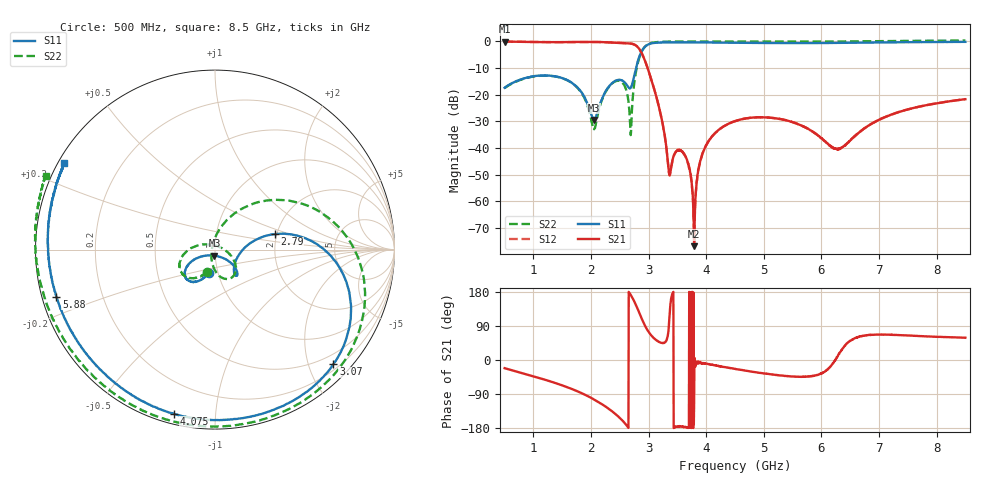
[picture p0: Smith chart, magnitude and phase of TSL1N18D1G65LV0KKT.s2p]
!TSL1N18D1G65LV0KKT  S-PARAMETER MODEL  ( General Type )
! Model Generated by TAIYO YUDEN Corporation (https://www.yuden.co.jp/en/)
! Version 1.0
! TAIYO YUDEN Control No. 240527
! Copyright(c) 2024 TAIYO YUDEN CO.,LTD. All Rights Reserved.
! Products Name : Ceramic RF Devices
! Characteristics :
!  Passband freq :617-2690MHz, , ( At Passband , Insertion Loss :1.35dB, VSWR 2.0 )
!  Attenuation :30 dB min at 3300 to 3800MHz,24 dB min at 4400to 7125MHz, Impedance : 50 Ohm
!  Case Size : 1.6 x 0.8 / 0.063 x 0.031 [mm/inch] , Thickness : 0.65 / 0.026 [mm/inch]
!  (Conditions: Temperature = 25 degC , DC Bias Current/Voltage = 0A / 0V)
! External Node Assignments :
!  1  o---|-------|---o  2
!  |  LPF  |
! GND o---|-------|---o GND
! Frequency Range : 500MHz  -  8.5GHz  [ 1601 STEP ]
# MHz S RI R 50
! Freq[MHz].  S11 Real  S11 Imag  S21 Real  S21 Imag  S12 Real  S12 Imag  S22 Real  S22 Imag
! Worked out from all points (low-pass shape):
!   1601 points, 500 MHz to 8.5 GHz, reference 50 ohm
!   highest |S21| = -0.15 dB at 500 MHz (marker M1); lowest = -76.8 dB at 3.79 GHz (marker M2)
!   |S21| within 3 dB of the highest: start of sweep to 2.845 GHz
!   lowest |S11| = -29.5 dB at 2.055 GHz (marker M3), VSWR 1.07, Z = 49.6 - j3.31 ohm
!   |S11| at or under -10 dB: start of sweep to 2.782 GHz
!   |S22| runs from -35.2 to 0.3 dB; largest |S21 - S12| = 0.0035
!   S11 on the Smith chart (normalised r, x): 500 MHz: 0.90, -0.24; 2.79 GHz: 1.95, +0.38; 3.07 GHz: 0.30, -2.44; 4.075 GHz: 0.05, -0.78; 5.88 GHz: 0.04, -0.14; 8.5 GHz: 0.02, +0.27
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500  -0.0351 -0.1294  0.9144 -0.3612  0.9142 -0.3619  -0.045 -0.1235
1280  -0.1622 -0.1571  0.5387 -0.7928  0.5377 -0.7915  -0.1935 -0.1141
1835  -0.0994 -0.0467  0.0446 -0.9672  0.0421 -0.9657  -0.1047 0.0206
2055  -0.00296 -0.0333  -0.2403 -0.938  -0.2411 -0.9365  0.00809 0.021
2430  0.1244 -0.1337  -0.7505 -0.5604  -0.7497 -0.5585  0.106 -0.1428
2580  0.1074 -0.1335  -0.8916 -0.2311  -0.8915 -0.2294  0.0239 -0.1471
2690  0.1305 -0.0342  -0.8932 0.1312  -0.8926 0.1331  -0.0172 0.00303
2790  0.3328 0.0864  -0.64 0.5042  -0.6389 0.5038  0.18 0.2417
2935  0.7481 -0.2366  -0.0102 0.436  -0.00937 0.4366  0.7859 -0.019
3070  0.6596 -0.6385  0.0773 0.1386  0.0779 0.1391  0.7712 -0.5324
3170  0.5185 -0.7863  0.0427 0.0483  0.0421 0.0489  0.6227 -0.7375
3355  0.2946 -0.904  -0.000484 0.00331  -0.000401 0.00336  0.3637 -0.9105
3615  0.0658 -0.9484  -0.00764 -0.000329  -0.00768 -0.000477  0.0948 -0.9799
3790  -0.059 -0.9475  -6.23e-05 -0.000131  9.43e-05 -0.000155  -0.0434 -0.985
3900  -0.1263 -0.938  0.00587 -0.00068  0.00579 -0.000702  -0.1179 -0.9784
4075  -0.2261 -0.9162  0.0147 -0.00325  0.0148 -0.0032  -0.2235 -0.9598
4500  -0.436 -0.8277  0.0293 -0.0126  0.0291 -0.0128  -0.4305 -0.8838
5835  -0.876 -0.2845  0.0153 -0.0139  0.0153 -0.014  -0.8608 -0.4694
5880  -0.8838 -0.2616  0.0146 -0.0127  0.0143 -0.0127  -0.8699 -0.4521
6305  -0.9263 -0.0478  0.00936 0.00282  0.00917 0.0026  -0.9464 -0.2776
7170  -0.9016 0.2927  0.0158 0.037  0.0161 0.037  -1 0.066
8500  -0.841 0.4843  0.0425 0.0702  0.0428 0.07  -0.9434 0.4124
